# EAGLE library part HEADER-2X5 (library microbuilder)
PIN HEADER
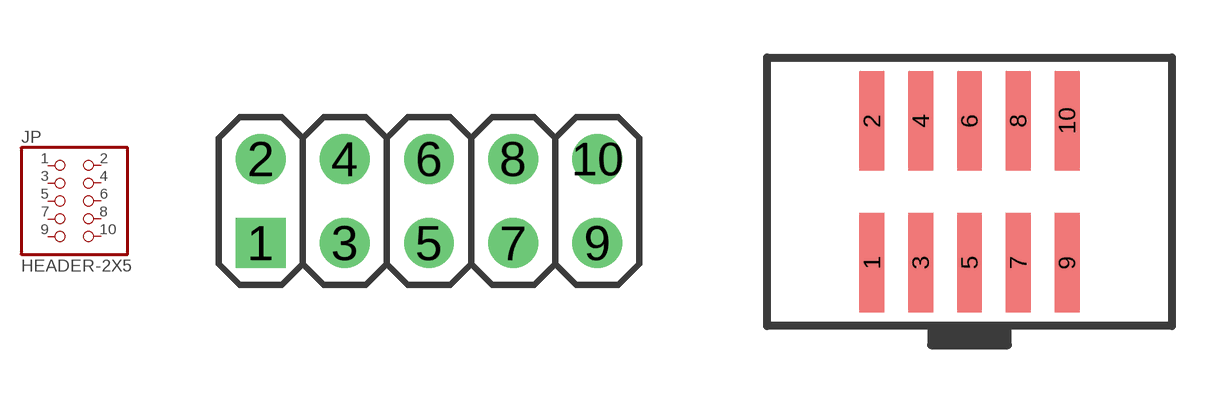
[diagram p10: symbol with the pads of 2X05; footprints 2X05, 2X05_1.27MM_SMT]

Designator prefix JP

## HEADER-2X5  [2X05]
1  1  pas
2  2  pas
3  3  pas
4  4  pas
5  5  pas
6  6  pas
7  7  pas
8  8  pas
9  9  pas
10  10  pas

## HEADER-2X51.27MM  [2X05_1.27MM_SMT]
Pads as for 2X05

## Footprint 2X05 (pad centres in mm)
PIN HEADER
drill 1 square: 1 -5.08,-1.27
drill 1: 2 -5.08,1.27; 3 -2.54,-1.27; 4 -2.54,1.27; 5 0,-1.27; 6 0,1.27; 7 2.54,-1.27; 8 2.54,1.27; 9 5.08,-1.27; 10 5.08,1.27

## Footprint 2X05_1.27MM_SMT (pad centres in mm)
2x05 1.27mm Headers SMT (2.0mm Height) 4UConnector: 16846
smd 0.65 x 2.6: 1 -2.54,-1.85; 2 -2.54,1.85; 3 -1.27,-1.85; 4 -1.27,1.85; 5 0,-1.85; 6 0,1.85; 7 1.27,-1.85; 8 1.27,1.85; 9 2.54,-1.85; 10 2.54,1.85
